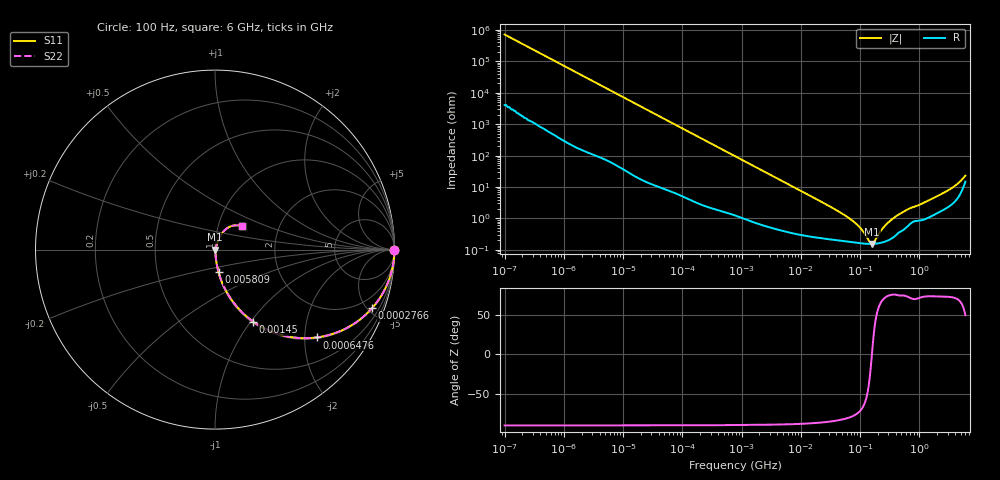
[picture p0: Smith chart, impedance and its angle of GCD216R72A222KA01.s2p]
!Murata Part Number: GCD216R72A222KA01
!These Parameters are Measured in Series Mode Connection
!Data Generated on Mar 13, 2026
!  o--ll--o
!Port1  Port2
!  o------o
!Operation Temp=25[degC], DC Bias Voltage=0[V]
!Freq. Start=100[Hz] Stop=6[GHz] 401[Steps]
# Hz S RI R 50
!Freq.(Hz) S11(Real) S11(Imag) S21(Real) S21(Imag) S12(Real) S12(Imag) S22(Real) S22(Imag)
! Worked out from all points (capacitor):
!   401 points, 100 Hz to 6 GHz, reference 50 ohm
!   read as one part in series: C = 2.21 nF near 109 Hz
!   lowest |Z| = 155 mohm at 159.6 MHz (marker M1)
!   series resonance near 158.5 MHz, so ESL is about 460 pH
!   S11 on the Smith chart (normalised r, x): 100 Hz: open; 276.6 kHz: 1.05, -5.34; 647.6 kHz: 1.03, -2.29; 1.45 MHz: 1.02, -1.03; 5.809 MHz: 1.01, -0.26; 6 GHz: 1.30, +0.35
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100  1 -0.000139  8e-07 0.000139  8e-07 0.000139  1 -0.000139
2008  1 -0.00276  1.91e-05 0.00276  1.91e-05 0.00276  1 -0.00276
40335  0.9967 -0.0548  0.00332 0.0548  0.00332 0.0548  0.9967 -0.0548
112960  0.976 -0.1496  0.024 0.1496  0.024 0.1496  0.976 -0.1496
276587  0.8749 -0.3266  0.1251 0.3266  0.1251 0.3266  0.8749 -0.3266
647581  0.5668 -0.4895  0.4332 0.4895  0.4332 0.4895  0.5668 -0.4895
774597  0.4794 -0.4931  0.5206 0.4931  0.5206 0.4931  0.4794 -0.4931
1449809  0.2133 -0.4019  0.7867 0.4019  0.7867 0.4019  0.2133 -0.4019
2594782  0.0814 -0.264  0.9186 0.264  0.9186 0.264  0.0814 -0.264
5809218  0.0201 -0.1268  0.9799 0.1268  0.9799 0.1268  0.0201 -0.1268
1.555665e7  0.00492 -0.0483  0.9951 0.0483  0.9951 0.0483  0.00492 -0.0483
7.129496e7  0.00184 -0.00885  0.9982 0.00885  0.9982 0.00885  0.00184 -0.00885
1.020051e8  0.00164 -0.00461  0.9984 0.00461  0.9984 0.00461  0.00164 -0.00461
1.459435e8  0.00154 -0.000846  0.9985 0.000846  0.9985 0.000846  0.00154 -0.000846
1.596157e8  0.00155 7.67e-05  0.9985 -7.67e-05  0.9985 -7.67e-05  0.00155 7.67e-05
1.745687e8  0.00156 0.00101  0.9984 -0.00101  0.9984 -0.00101  0.00156 0.00101
2.388273e8  0.00174 0.0044  0.9983 -0.0044  0.9983 -0.0044  0.00174 0.0044
3.124326e8  0.00215 0.00768  0.9979 -0.00768  0.9979 -0.00768  0.00215 0.00768
6.11557e8  0.00558 0.0178  0.9944 -0.0178  0.9944 -0.0178  0.00558 0.0178
3.065283e9  0.0277 0.0713  0.9723 -0.0713  0.9723 -0.0713  0.0277 0.0713
4.586474e9  0.0595 0.1129  0.9405 -0.1129  0.9405 -0.1129  0.0595 0.1129
6e9  0.1489 0.1297  0.8511 -0.1297  0.8511 -0.1297  0.1489 0.1297
